PROGRAM MAIN
VAR
	random1				:	ARRAY [1..MAX(2,randomnum)] OF random_dice;
	randomtime			:	ARRAY [1..MAX(2,randomnum)] OF random_time;
	start				:	BOOL;
	estart				:	BOOL;
	stop				:	BOOL;
	estop				:	BOOL;
	done				:	ARRAY[1..MAX(2,randomnum)] OF BOOL;
	HMILampState		:	ARRAY[1..MAX(2,randomnum)] OF LampState;
	
	eachdata			:	ARRAY[1..MAX(2,randomnum)] OF UINT := [3(1)];
	aPoints 			: 	ARRAY[1..2,0..400] OF ST_Point;
	PT					:	ARRAY[1..MAX(2,randomnum)] OF  TIME;
	invisible			:	ARRAY[1..MAX(2,randomnum)] OF ARRAY[1..6] OF BOOL;
	bvisiable : int; // 测试用变量
	
	//twincat hmi visible
	visible				:	ARRAY[1..MAX(2,randomnum)] OF ARRAY[1..6] OF STRING;
	
	totalscore			:	UINT;
	totalscorebuffer 	:	ARRAY [0..65535]OF UINT;
	record1				:	ARRAY [0..65535]OF record;
	HMIShowrecord		:	ARRAY [0..400]OF record;
	
	counter				:	UINT;
		
	seed				:	ARRAY[1..3] OF INT := [27000, 24000, 32000];
	i					:	UINT;
	ton1				:	ARRAY [1..3] OF TON;
	tontemp				:	ton;
	
	doneRtrig			:	ARRAY [1..3] OF R_trig;	
	ftrigstop			:	f_trig;
	rtrigstart			:	R_trig;
	rtrigstart1			:	R_trig;
	

	
	FBGetTime			:	NT_GetTime;
	FBLocalSystemTime	:	FB_LocalSystemTime;
	bSystemTimeEnable	:	BOOL;
	systemTime			:	TIMESTRUCT;
	systemTimeString	:	STRING;
	eachDataString		:	STRING;
	scoreStateString	:	WSTRING;
	stateResult			:	WSTRING;
	nameOfScore			:	WSTRING;
	
	
	FB_FormatString1	:	FB_FormatString;
	FB_FormatString2	:	FB_FormatString;
	FB_FormatString3	:	FB_FormatString;
	
	
	gamestate			:	INT;

	donecounterRtrig	:	R_trig;
	b1					:	BOOL;
	GetTimeTon			:	Ton;
	nCounter			:	UINT;
	vCounter			:	UINT;
	xaxismin			:	UINT;
	xaxismax			:	UINT:=1;
	
	
	HMIBigCounter		:	UINT;
	HMILitterCounter	:	UINT;
	HMIALLWIN			:	UINT;
	HMIEqual			:	UINT;
END_VAR


VAR CONSTANT
	randomnum: UINT:=3;//骰子个数
END_VAR

// 使用本样例程序，仅需要激活配置并login程序即可，HMI界面的部分，可以使用Live View功能来预览，也可以发布到本机直接使用
// 使用TwinCAT 3编写程序，使用随机数实现投三个骰子小程序，让玩家们猜大小，同时提供历史记录以及数据统计的功能。

CASE gamestate OF 
	// 游戏主进程
	0:  
		// PLC主进程中，当HMI中的开始按钮被按下，则触发骰子旋转的逻辑，将所有功能块复位
		rtrigstart(CLK:= start, Q=> );
		IF rtrigstart.Q THEN
			estart:=TRUE;
			FOR i:=1 TO 3 DO
				randomtime[i].start:=FALSE;
				random1[i].start:=FALSE;

			END_FOR
			
			// 跳转至下一阶段
			gamestate:=1;
		END_IF
		
	1:
		// 启动所有骰子，触发所有随机数，骰子开始转动，等待停止按钮触发
		FOR i:=1 TO 3 DO
			randomtime[i].start:=TRUE;
			random1[i].start:=TRUE;
		END_FOR
		

		// 所有骰子停止
		IF ton1[3].Q THEN
			estart:=FALSE;
			gamestate:=0;
		END_IF
		
bvisiable := bvisiable + 1;
	
END_CASE

// 骰子相关的功能块配置在ACT_Random这个action中，使用了本程序中封装的random_dice以及random_time功能块实现
ACT_Random();
// HMI界面显示
ACT_HMI_LAMP();
// 获取当前系统时间
Act_getSystemTime();
// 根据点数判断最终结果（大，小，豹子等）
Act_scoreState();
// 字符拼接，在界面上显示时间等信息
Act_usingFormatString();
// 统计结果的总数，生成图标输出到界面上
Act_console();
// 定时器，提供三个骰子的停转时间，第一个骰子先停止，第二个其次，第三个最后
ACT_time_trig();

ACTION Act_console:
// 每一次的游戏结果写入到数组中进行总和统计，生成各类结果的统计数量，配合HMI界面显示出来


donecounterRtrig(CLK:=random1[3].done);


IF donecounterRtrig.Q THEN

	IF counter < 0 OR counter > 65535 THEN
		counter:= 0;
	END_IF	  			
	totalscorebuffer[counter]				:=	totalscore;
	record1[counter].counter				:=	counter;
	record1[counter].localSystemTime		:=	systemTimeString;
	record1[counter].totalScore				:=	UINT_TO_STRING(totalscore);	
	//stateResult:=WCONCAT(nameOfScore,",");
	//stateResult:=WCONCAT(stateResult,scoreStateString);
	record1[counter].scoreState				:=	stateResult;
	record1[counter].threeEachPoint			:=	eachDataString;
	counter:= counter + 1;
	
	
	CASE totalscore OF
	4,5,6,7,8,9,10:
		HMILitterCounter :=HMILitterCounter	+	1;
	
	;
	
	
	11,12,13,14,15,17:
		HMIBigCounter	:=HMIBigCounter	+	1;
	;


	3,18:
		HMIALLWIN		:=HMIALLWIN	+	1;
	END_CASE
	
	
	IF eachdata[1] = eachdata[2] AND eachdata[2] = eachdata[3] THEN
		HMIEqual	:=HMIEqual	+1;	
	END_IF

	
	ACT_HMI_Chart();


END_IF
END_ACTION

ACTION Act_getSystemTime:
(*FBLocalSystemTime(
	sNetID:= '', 
	bEnable:= bSystemTimeEnable, 
	dwCycle:= 1, 
	dwOpt:= , 
	tTimeout:= , 
	bValid=> , 
	systemTime=> systemTime, 
	tzID=> );*)

GetTimeTon(IN:= NOT GetTimeTon.Q, PT:= T#500MS, Q=> , ET=> );

	
FBGetTime(
	NETID:= '', 
	START:= GetTimeTon.Q, 
	TMOUT:= , 
	BUSY=> , 
	ERR=> , 
	ERRID=> , 
	TIMESTR=> systemTime);
END_ACTION

ACTION ACT_HMI_Chart:
//坐标共计400个点，上万个点容易把twincathmi卡住

FOR nCounter := 0 TO 400 DO

		aPoints[1, nCounter].x := nCounter;
		
		// graph 2 单根线10.5
		aPoints[2, nCounter].x := nCounter;
		aPoints[2, nCounter].y := 10.5;
END_FOR

IF vCounter	>20 THEN
	xaxismin	:=	xaxismin	+	1;
	//xaxismax	:=	xaxismax	+	1;
END_IF

IF vCounter	>400 THEN
	vCounter	:=	0;
END_IF

//aPoints[1, vCounter].y := UINT_TO_LREAL(totalscore);	

//历史表格一起写过来

	HMIShowrecord[vCounter].counter				:=	counter;
	HMIShowrecord[vCounter].localSystemTime		:=	systemTimeString;
	HMIShowrecord[vCounter].totalScore				:=	UINT_TO_STRING(totalscore);	
	HMIShowrecord[vCounter].scoreState				:=	stateResult;
	HMIShowrecord[vCounter].threeEachPoint			:=	eachDataString;

//twincat hmi xychart 横坐标范围显示
//vCounter计数
vCounter	:=	vCounter	+	1;

IF vCounter > 1 THEN
	//xaxismin	:=	xaxismin	+	1;
	xaxismax	:=	xaxismax	+	1;
END_IF


(*IF vCounter = 1 THEN
	xaxismin	:=	xaxismin	+	1;
END_IF*)


FOR	nCounter:=vcounter	TO	400	BY	1	DO 
	aPoints[1,nCounter].y := UINT_TO_LREAL(totalscore);
END_FOR
END_ACTION

ACTION ACT_HMI_LAMP:
(*通过切换亮和灭两张图片，实现小灯点亮和灭灯的效果*)
FOR i:=1 TO 3 BY 1 DO
	
	IF done[i] THEN
		HMILampState[i].ON	:= 	'Visible';
		HMILampState[i].OFF	:= 	'Hidden';
	ELSE
		HMILampState[i].ON	:= 	'Hidden';
		HMILampState[i].OFF	:= 	'Visible';
	
	END_IF	
END_FOR
END_ACTION

ACTION ACT_Random:
FOR i:=1 TO 3 DO
	randomtime[i](
		start:= , 
		Seed:= Seed[i], 
		stop:= estop, 
		buffer=>,
		PT=> PT);


	random1[i](
		start:= , 
		Seed:= Seed[i], 
		stop:= ton1[i].Q, 
		//buffer=> buffer[i],
		invisible=>invisible[i],
		visible=>visible[i],
		data=> eachdata[i],
		done=>	done[i]);
	
	totalscore:= eachdata[1] + eachdata[2] + eachdata[3];	

END_FOR
END_ACTION

ACTION Act_scoreState:
(*得到三个骰子的结果计算总和之后，Act_scoreState中根据算得的结果，输出文字“大”，“小”，“全赢”等，显示在配套界面上*)
CASE totalscore OF
	4,5,6,7,8,9,10:
		scoreStateString:="小";
	
	;
	
	
	11,12,13,14,15,17:
		scoreStateString:="大";
	;


	3:
		scoreStateString:="围一";
		nameOfScore:="全赢";
		
	18:
		scoreStateString:="围六";
		nameOfScore:="全赢";

;

END_CASE

IF eachdata[1] = eachdata[2] AND eachdata[2] = eachdata[3] THEN
	nameOfScore:="豹子";
	ELSE
	nameOfScore:="";	
END_IF




//stateResult:=scoreStateString;
IF NOT (nameOfScore="") THEN
	stateResult:=WCONCAT(nameOfScore,",");
	stateResult:=WCONCAT(stateResult,scoreStateString);
ELSE
	stateResult:=scoreStateString;
END_IF
END_ACTION

ACTION ACT_time_trig:
(*当触发停止按钮后，将会触发ACT_time_trig这个ACTION中的3个定时器，
三个定时器分别设置了不同的延时时间，以达到3个骰子依次停转的效果。*)
ftrigstop(CLK:=stop);
	IF ftrigstop.Q THEN
		estop:=TRUE;
	END_IF
	


	ton1[1](IN:=estop , PT:=PT[1] , Q=> , ET=> );
	ton1[2](IN:=estop , PT:=PT[2] , Q=> , ET=> );
	ton1[3](IN:=estop , PT:=PT[3] , Q=> , ET=> );
	
	IF ton1[3].Q THEN
		estop:=FALSE;
	END_IF
END_ACTION

ACTION Act_usingFormatString:
FB_FormatString1(
	sFormat:= '%d-%d-%d %d:%d:%d', 
	arg1:=  F_WORD(systemTime.wYear), 
	arg2:=  F_WORD(systemTime.wMonth), 
	arg3:=  F_WORD(systemTime.wDay), 
	arg4:=  F_WORD(systemTime.wHour), 
	arg5:=  F_WORD(systemTime.wMinute), 
	arg6:=  F_WORD(systemTime.wSecond), 
	arg7:=  , 
	arg8:= , 
	arg9:= , 
	arg10:= , 
	bError=> , 
	nErrId=> , 
	sOut=> systemTimeString);
	
	
FB_FormatString2(
	sFormat:= '%d , %d , %d', 
	arg1:=  F_UINT(eachdata[1]), 
	arg2:=  F_UINT(eachdata[2]), 
	arg3:=  F_UINT(eachdata[3]), 
	arg4:=  , 
	arg5:=  , 
	arg6:=  , 
	arg7:=  ,
	arg8:= , 
	arg9:= , 
	arg10:= , 
	bError=> , 
	nErrId=> , 
	sOut=> eachDataString);
END_ACTION

END_PROGRAM
